FUNCTION_BLOCK FB 10
TITLE =
VERSION : 0.1


VAR_INPUT
  S1 : BOOL ;
  _1B1 : BOOL ;
  _1B2 : BOOL ;
  _2B1 : BOOL ;
  _2B2 : BOOL ;
  _3B1 : BOOL ;
  _3B2 : BOOL ;
  Zeit : TIMER ;
  Zeitw : S5TIME ;
  RESET : BOOL ;
END_VAR
VAR_OUTPUT
  _1Y1 : BOOL ;
  _1Y2 : BOOL ;
  _2Y1 : BOOL ;
  _3Y1 : BOOL ;
END_VAR
VAR
  SRO_1 : BOOL  := TRUE;
  SRO_2 : BOOL ;
  SRO_3 : BOOL ;
  SRO_4 : BOOL ;
  SRO_5 : BOOL ;
  SRO_6 : BOOL ;
  SRO_7 : BOOL ;
END_VAR
BEGIN
NETWORK
TITLE =
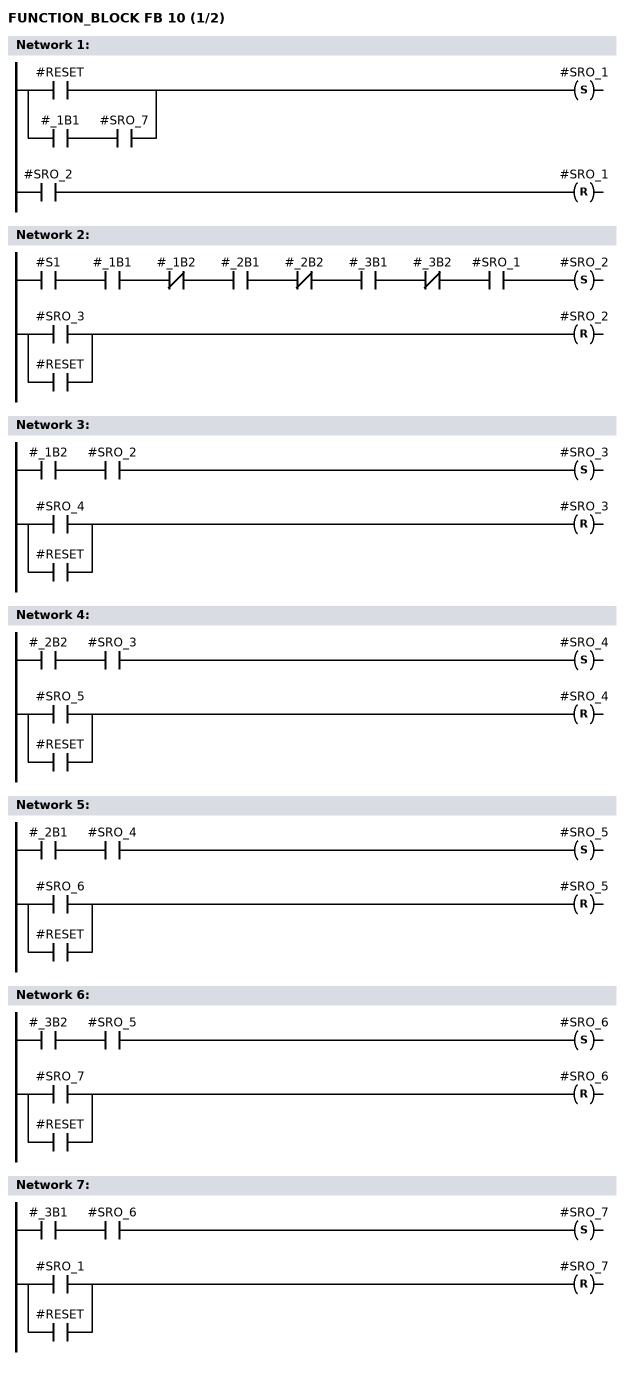
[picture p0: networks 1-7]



      U(    ;
      O     #RESET;
      O     ;
      U     #_1B1;
      U     #SRO_7;
      )     ;
      S     #SRO_1;
      U     #SRO_2;
      R     #SRO_1;
      NOP   0;
NETWORK
TITLE =

      U     #S1;
      U     #_1B1;
      UN    #_1B2;
      U     #_2B1;
      UN    #_2B2;
      U     #_3B1;
      UN    #_3B2;
      U     #SRO_1;
      S     #SRO_2;
      U(    ;
      O     #SRO_3;
      O     #RESET;
      )     ;
      R     #SRO_2;
      NOP   0;
NETWORK
TITLE =

      U     #_1B2;
      U     #SRO_2;
      S     #SRO_3;
      U(    ;
      O     #SRO_4;
      O     #RESET;
      )     ;
      R     #SRO_3;
      NOP   0;
NETWORK
TITLE =

      U     #_2B2;
      U     #SRO_3;
      S     #SRO_4;
      U(    ;
      O     #SRO_5;
      O     #RESET;
      )     ;
      R     #SRO_4;
      NOP   0;
NETWORK
TITLE =

      U     #_2B1;
      U     #SRO_4;
      S     #SRO_5;
      U(    ;
      O     #SRO_6;
      O     #RESET;
      )     ;
      R     #SRO_5;
      NOP   0;
NETWORK
TITLE =

      U     #_3B2;
      U     #SRO_5;
      S     #SRO_6;
      U(    ;
      O     #SRO_7;
      O     #RESET;
      )     ;
      R     #SRO_6;
      NOP   0;
NETWORK
TITLE =

      U     #_3B1;
      U     #SRO_6;
      S     #SRO_7;
      U(    ;
      O     #SRO_1;
      O     #RESET;
      )     ;
      R     #SRO_7;
      NOP   0;
NETWORK
TITLE =
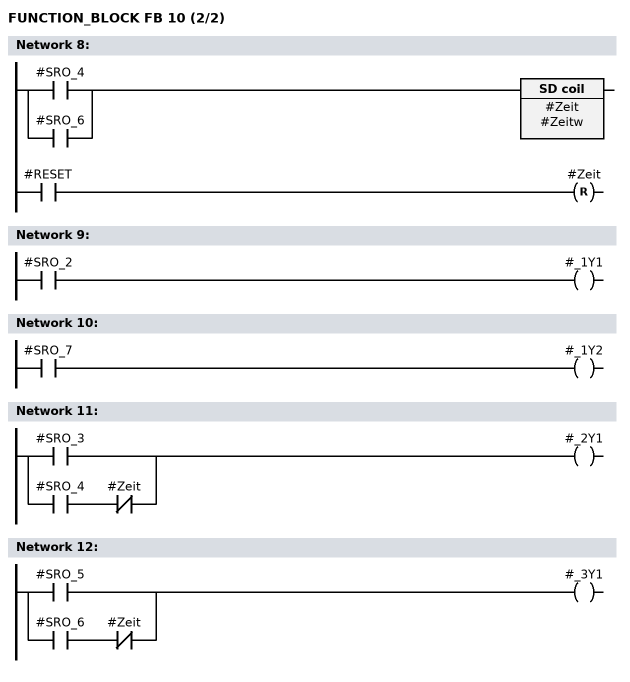
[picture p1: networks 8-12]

      U(    ;
      O     #SRO_4;
      O     #SRO_6;
      )     ;
      L     #Zeitw;
      SE    #Zeit;
      U     #RESET;
      R     #Zeit;
      NOP   0;
      NOP   0;
      NOP   0;
NETWORK
TITLE =

      U     #SRO_2;
      =     #_1Y1;
NETWORK
TITLE =

      U     #SRO_7;
      =     #_1Y2;
NETWORK
TITLE =

      O     #SRO_3;
      O     ;
      U     #SRO_4;
      UN    #Zeit;
      =     #_2Y1;
NETWORK
TITLE =

      O     #SRO_5;
      O     ;
      U     #SRO_6;
      UN    #Zeit;
      =     #_3Y1;
END_FUNCTION_BLOCK

DATA_BLOCK DB 10
TITLE =
VERSION : 0.0

 FB 10
BEGIN
   S1 := FALSE;
   _1B1 := FALSE;
   _1B2 := FALSE;
   _2B1 := FALSE;
   _2B2 := FALSE;
   _3B1 := FALSE;
   _3B2 := FALSE;
   Zeit := T 0;
   Zeitw := S5T#0MS;
   RESET := FALSE;
   _1Y1 := FALSE;
   _1Y2 := FALSE;
   _2Y1 := FALSE;
   _3Y1 := FALSE;
   SRO_1 := TRUE;
   SRO_2 := FALSE;
   SRO_3 := FALSE;
   SRO_4 := FALSE;
   SRO_5 := FALSE;
   SRO_6 := FALSE;
   SRO_7 := FALSE;
END_DATA_BLOCK

